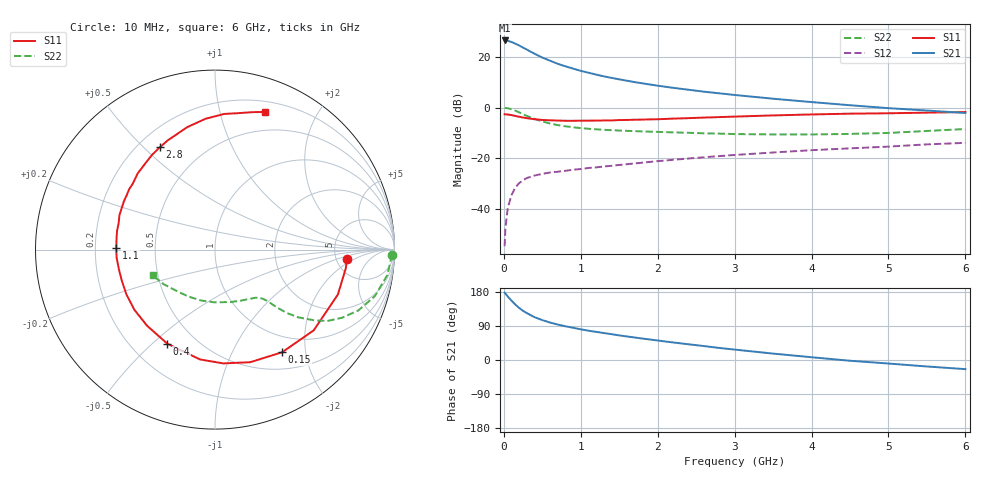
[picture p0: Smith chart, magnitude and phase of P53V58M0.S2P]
! SIEMENS Small Signal Semiconductors
! BFP183
! Si NPN RF Bipolar Junction Transistor in SOT143
! VCE = 3.5 V  IC = 8 mA
! Common Emitter S-Parameters:  March  1996
# GHz  S  MA  R  50
!  f  S11  S21  S12  S22
! GHz  MAG  ANG  MAG  ANG  MAG  ANG  MAG  ANG
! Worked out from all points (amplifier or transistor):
!   36 points, 10 MHz to 6 GHz, reference 50 ohm
!   highest |S21| = 26.6 dB at 10 MHz (marker M1)
!   |S21| within 3 dB of that: start of sweep to 259.5 MHz
!   unconditionally stable (mu >= 1): 1.293 GHz to 5.585 GHz
!   at 250 MHz: K = 0.28, MSG = 26.3 dB, |S12| = -28.8 dB
!   at 1.4 GHz: K = 1.04, MAG = 16.1 dB, |S12| = -23.1 dB
!   at 6 GHz: K = 0.94, MSG = 5.9 dB, |S12| = -14.0 dB
!   lowest NFmin = 1.30 dB at 450 MHz
!   S11 on the Smith chart (normalised r, x): 10 MHz: 6.29, -1.42; 150 MHz: 0.74, -1.59; 400 MHz: 0.35, -0.56; 1.1 GHz: 0.29, +0.01; 2.8 GHz: 0.29, +0.56; 6 GHz: 0.30, +1.39
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0.01  0.7376 -4.0  21.35 177.6  0.0018 81.4  0.9886 -1.7
0.02  0.7362 -8.1  21.32 175.4  0.004 83.4  0.9812 -3.4
0.05  0.729 -20.1  21 167.8  0.0101 81.6  0.9707 -8.4
0.1  0.7105 -39.3  19.87 156.5  0.0185 71.6  0.9272 -16.3
0.15  0.6834 -56.8  18.44 146.1  0.0263 63.4  0.8674 -23.0
0.2  0.6575 -72.6  16.97 137.3  0.032 57.8  0.8034 -28.2
0.25  0.6357 -85.9  15.38 129.7  0.0364 52.8  0.7419 -32.4
0.3  0.6176 -97.8  14.04 123.6  0.0403 49.4  0.6834 -35.3
0.4  0.5876 -116.9  11.63 113.0  0.0451 43.9  0.5966 -39.2
0.5  0.5685 -131.7  9.78 105.2  0.0487 40.6  0.5318 -41.5
0.6  0.5606 -143.3  8.493 98.9  0.0518 39.2  0.4839 -42.7
0.7  0.5531 -153.2  7.368 93.6  0.0537 38.6  0.45 -43.5
0.9  0.5467 -168.4  5.912 85.1  0.0588 38.0  0.4076 -44.5
1.1  0.5504 179.1  4.901 77.3  0.0636 38.5  0.3802 -46.0
1.5  0.5658 160.3  3.626 64.9  0.073 39.3  0.3508 -49.9
1.8  0.5778 148.4  3.024 56.6  0.081 39.6  0.3371 -54.1
2.2  0.6047 135.4  2.462 46.3  0.0924 39.5  0.323 -60.7
2.8  0.6476 118.4  1.917 31.8  0.1094 37.3  0.3053 -73.2
3.5  0.6995 102.8  1.498 16.9  0.129 34.0  0.2939 -90.5
4.5  0.7576 86.1  1.113 -2.0  0.1558 27.5  0.3009 -119.8
5.5  0.7935 74.8  0.874 -17.1  0.1867 21.3  0.3445 -145.8
6  0.8166 69.9  0.781 -24.1  0.2002 17.0  0.3761 -157.5
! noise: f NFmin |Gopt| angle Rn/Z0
0.45  1.3  0.17  43  0.21
0.9  1.35  0.21  115  0.2
1.8  2.05  0.33  -177  0.14
